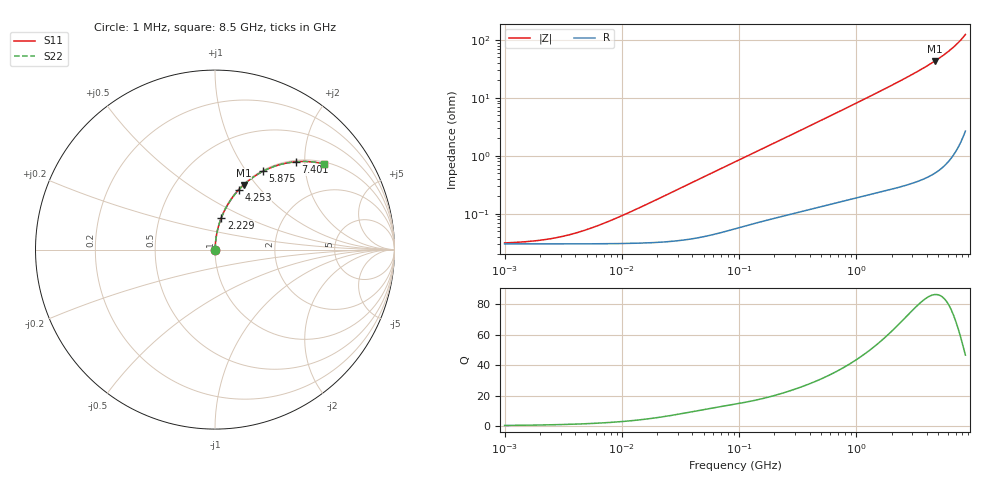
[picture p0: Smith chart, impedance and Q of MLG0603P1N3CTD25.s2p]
! S-Parameter Data Generated by TDK Corporation
! Copyright(C) 2025 TDK Corporation.
! All Rights Reserved.
! TDK P/N: MLG0603P1N3CTD25 (SMD / SMT Inductor (Coil))
! Property: L=1.3nH at 500MHz
! Size(LxWxT): 0.6x0.3x0.3mm
! Model Type: s2p (Touchstone File Format Version 1.0)
! Frequency: DC=Yes Start=1MHz Stop=8500MHz 198points Log-sweep
! Model Generated on Feb. 6, 2025
! Terms and conditions regarding TDK Simulation Models:
! 1)This simulation model is being provided solely for informational
!  purposes. Please refer to the specifications of the products in
!  terms of detailed characteristics of such products.
! 2)In no event shall TDK Corporation of any of its subsidiaries be
!  liable for any loss or damage arising, directly or indirectly,
!  from any information contained in this simulation model, including,
!  but not limited to loss or damages arising from any inaccuracies,
!  omissions or errors in connection with such information.
! 3)Any and all copyrights on this simulation model are owned by
!  TDK Corporation.  Duplication or redistribution of this simulation
!  model without prior written permission from TDK Corporation
!  is prohibited.
! 4)This simulation model is subject to any modification or change
!  without any prior notice.
! 5)Neither TDK Corporation nor any of its subsidiaries shall make any
!  warranty, express or implied, including but not limited to the
!  correctness, implied warranties of merchantability and fitness for
!  a particular purpose with respect to this simulation models.
! 6)The use of this simulation model shall be deemed to have consented
!  to the terms and conditions hereof.
! Port Assignments:
!  1 ---@@@--- 2
! Applicable Conditions:
!  Temperature = 25 degC
!  DC Bias Current = 0 A
!  Small Signal Operation
# Hz S MA R 50
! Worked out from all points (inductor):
!   197 points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, 1 MHz to 8.5 GHz, reference 50 ohm
!   read as one part in series: L = 1.38 nH near 11.03 MHz
!   highest Q = 86.4 at 4.664 GHz (marker M1), where L = 1.47 nH
!   S11 on the Smith chart (normalised r, x): 1 MHz: 1.00, +0.00; 2.229 GHz: 1.01, +0.37; 4.253 GHz: 1.01, +0.77; 5.875 GHz: 1.01, +1.20; 7.401 GHz: 1.03, +1.80; 8.5 GHz: 1.05, +2.49
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1000000  0.0003123 16.2  0.9997 -0.0  0.9997 -0.0  0.0003123 16.2
1586648  0.0003302 24.7  0.9997 -0.0  0.9997 -0.0  0.0003302 24.7
2295435  0.0003605 33.6  0.9997 -0.0  0.9997 -0.0  0.0003605 33.6
3320851  0.0004167 43.9  0.9997 -0.0  0.9997 -0.0  0.0004167 43.9
4587603  0.0004997 52.9  0.9997 -0.0  0.9997 -0.0  0.0004997 52.9
6337562  0.0006283 61.3  0.9997 -0.0  0.9997 -0.0  0.0006283 61.3
8755050  0.0008195 68.2  0.9997 -0.0  0.9997 -0.0  0.0008195 68.2
2.10461e7  0.001854 79.9  0.9997 -0.1  0.9997 -0.1  0.001854 79.9
9.219544e7  0.007843 85.6  0.9994 -0.4  0.9994 -0.4  0.007843 85.6
4.229561e8  0.03459 86.0  0.9982 -2.0  0.9982 -2.0  0.03459 86.0
1.016736e9  0.08223 84.0  0.9947 -4.7  0.9947 -4.7  0.08223 84.0
1.940355e9  0.1571 80.0  0.985 -9.0  0.985 -9.0  0.1571 80.0
2.228565e9  0.1809 78.7  0.9808 -10.4  0.9808 -10.4  0.1809 78.7
3.224109e9  0.2652 73.9  0.9608 -15.4  0.9608 -15.4  0.2652 73.9
4.253027e9  0.3566 68.4  0.9301 -20.9  0.9301 -20.9  0.3566 68.4
4.664383e9  0.3946 66.1  0.9143 -23.2  0.9143 -23.2  0.3946 66.1
5.357206e9  0.4605 61.9  0.8823 -27.4  0.8823 -27.4  0.4605 61.9
5.87536e9  0.5112 58.6  0.8533 -30.7  0.8533 -30.7  0.5112 58.6
6.748056e9  0.5985 52.5  0.793 -36.8  0.793 -36.8  0.5985 52.5
7.400733e9  0.6642 47.5  0.7372 -41.6  0.7372 -41.6  0.6642 47.5
8.116539e9  0.7348 41.6  0.6644 -47.3  0.6644 -47.3  0.7348 41.6
8.5e9  0.7712 38.3  0.6202 -50.4  0.6202 -50.4  0.7712 38.3
